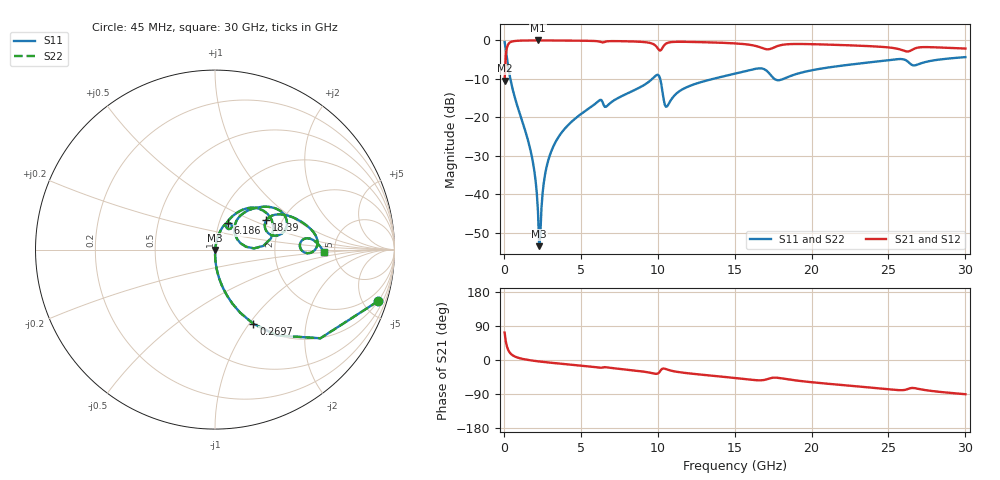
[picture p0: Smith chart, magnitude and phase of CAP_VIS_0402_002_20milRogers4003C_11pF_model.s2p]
! S-parameter model data by Modelithics Inc.  support@modelithics.com  813-866-6335  Tampa FL USA
! S-Parameter data specifications:
! Substrate: 20-mil Rogers 4003C, substrate thickness, H=0.508mm, Dielectric constant, Er=3.75
! PCB Mounting Pad Footprint: Pad width, PadW=0.50mm , Pad length, PadL=0.50mm , Pad gap, PadG (edge-to-edge)=0.40mm , Reference planes=1.4mm apart
! Created Wed Nov 18 12:51:18 2015
# hz S ma R 50
! 2 Port Network Data from SP1.SP block
! freq  magS11  angS11  magS21  angS21  magS12  angS12  magS22  angS22
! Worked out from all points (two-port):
!   401 points, 45 MHz to 30 GHz, reference 50 ohm
!   highest |S21| = -0.01 dB at 2.217 GHz (marker M1); lowest = -10.5 dB at 45 MHz (marker M2)
!   |S21| within 3 dB of the highest: 151.9 MHz to end of sweep
!   lowest |S11| = -53.5 dB at 2.292 GHz (marker M3), VSWR 1.00, Z = 50.1 - j0.16 ohm
!   |S11| at or under -10 dB: 417.8 MHz to 9.647 GHz (9.229 GHz wide, 183 % of centre); 10.16 GHz to 13.6 GHz (3.444 GHz wide, 29 % of centre); 17.58 GHz to 18.18 GHz (597.7 MHz wide, 3.34 % of centre)
!   |S22| runs from -53.5 to -0.4 dB; largest |S21 - S12| = 0
!   S11 on the Smith chart (normalised r, x): 45 MHz: 0.99, -6.37; 269.7 MHz: 0.99, -1.05; 6.186 GHz: 1.10, +0.34; 18.39 GHz: 1.66, +0.61; 30 GHz: 4.07, -0.17
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4.5e7  0.9544 -17.4  0.2985 72.6  0.2985 72.6  0.9544 -17.4
2.696625e8  0.4658 -62.6  0.8844 27.3  0.8844 27.3  0.4658 -62.6
6.441e8  0.202 -79.2  0.9786 10.5  0.9786 10.5  0.202 -79.2
1.767412e9  0.03427 -88.9  0.9981 -1.1  0.9981 -1.1  0.03427 -88.9
1.992075e9  0.01909 -88.2  0.9984 -2.3  0.9984 -2.3  0.01909 -88.2
2.216738e9  0.005835 -79.1  0.9985 -3.5  0.9985 -3.5  0.005835 -79.1
2.291625e9  0.002106 -49.3  0.9985 -3.8  0.9985 -3.8  0.002106 -49.3
2.4414e9  0.006595 72.1  0.9984 -4.6  0.9984 -4.6  0.006595 72.1
2.74095e9  0.02109 79.7  0.9981 -5.9  0.9981 -5.9  0.02109 79.7
3.115388e9  0.03768 79.9  0.9975 -7.5  0.9975 -7.5  0.03768 79.9
5.062462e9  0.1121 73.5  0.9909 -15.1  0.9909 -15.1  0.1121 73.5
6.185775e9  0.1648 63.9  0.969 -20.0  0.969 -20.0  0.1648 63.9
9.6306e9  0.314 48.0  0.9099 -34.7  0.9099 -34.7  0.314 48.0
1.007992e10  0.3473 19.8  0.7523 -33.4  0.7523 -33.4  0.3473 19.8
1.060414e10  0.1384 34.5  0.9223 -25.0  0.9223 -25.0  0.1384 34.5
1.187722e10  0.2459 52.7  0.9575 -34.6  0.9575 -34.6  0.2459 52.7
1.50225e10  0.3697 40.2  0.914 -47.5  0.914 -47.5  0.3697 40.2
1.68198e10  0.4288 20.8  0.7927 -53.3  0.7927 -53.3  0.4288 20.8
1.839244e10  0.3295 29.8  0.8902 -50.6  0.8902 -50.6  0.3295 29.8
2.003996e10  0.4097 28.6  0.8931 -58.8  0.8931 -58.8  0.4097 28.6
2.505742e10  0.5556 10.3  0.8083 -77.4  0.8083 -77.4  0.5556 10.3
3e10  0.6062 -1.2  0.7838 -90.3  0.7838 -90.3  0.6062 -1.2
